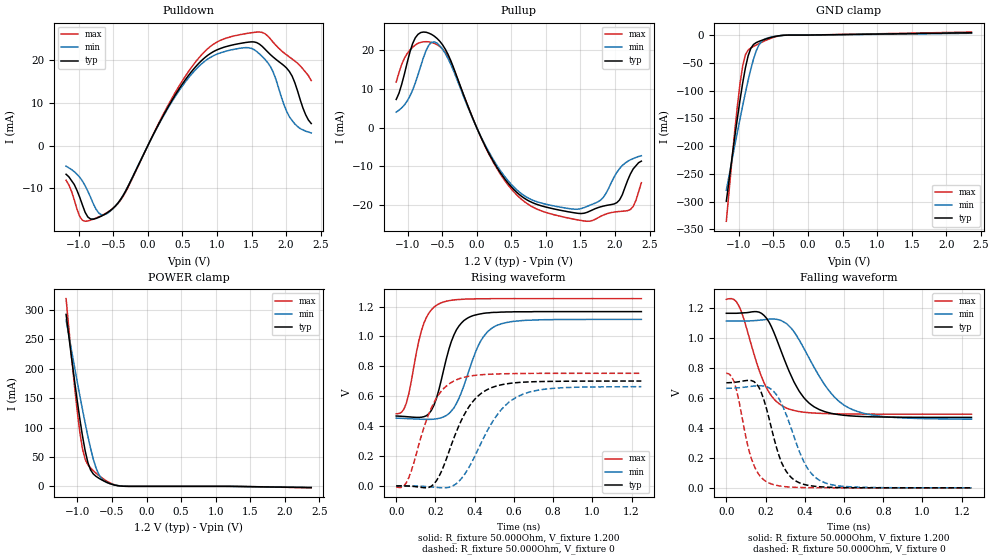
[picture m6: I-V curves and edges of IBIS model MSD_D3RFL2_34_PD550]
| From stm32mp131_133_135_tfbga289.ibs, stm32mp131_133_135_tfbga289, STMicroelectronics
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[Model] MSD_D3RFL2_34_PD550
Model_type   I/O
C_comp 2.431pF   2.345pF   2.556pF
Vinh = 820.000mV
Vinl = 380.000mV
Vmeas = 600.000mV
Vref = 600.000mV
[Model Spec]
Vinh   820.000mV   790.000mV   870.000mV
Vinl   380.000mV   350.000mV   430.000mV
Vmeas   600.000mV   570.000mV   650.000mV
Vref   600.000mV   570.000mV   650.000mV
[Receiver Thresholds]
Vth   =  0.600V
Vth_min  =  0.5880V
Vth_max  =  0.6120V
Vinh_ac  =  0.220V
Vinh_dc  =  0.130V
Vinl_ac  = -0.220V
Vinl_dc  = -0.130V
Tslew_ac =  5.000ns |Not specified, so set to high value
[Temperature Range]   25.000   125.000   -40.000
[Voltage Range]   1.200V   1.140V   1.300V
[GND Clamp Reference]   0.00V   0.00V   0.00V
[Pulldown Reference]   0.00V   0.00V   0.00V
[POWER Clamp Reference]   1.200V   1.140V   1.300V
[Pullup Reference]   1.200V   1.140V   1.300V
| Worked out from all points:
|   slope of the pulldown table from 0 to 0.18 V, typ, clamps not added: 31.3 ohm
|   slope of the pullup table from 0 to 0.18 V, typ, clamps not added: 26.5 ohm
|   GND clamp passes 1 mA (typ) near -0.40 V on its own axis
|   POWER clamp passes 1 mA (typ) near -0.41 V on its own axis
|   rising waveform, R_fixture 50.000Ohm, V_fixture 1.200: 20-80 % time 90.7ps typ, 117ps min, 77.4ps max; typ from 0.468 V to 1.17 V
|   rising waveform, R_fixture 50.000Ohm, V_fixture 0: 20-80 % time 145ps typ, 176ps min, 124ps max; typ from 0.001 V to 0.702 V
|   falling waveform, R_fixture 50.000Ohm, V_fixture 1.200: 20-80 % time 145ps typ, 191ps min, 120ps max; typ from 1.17 V to 0.47 V
|   falling waveform, R_fixture 50.000Ohm, V_fixture 0: 20-80 % time 94.7ps typ, 121ps min, 80.9ps max; typ from 0.701 V to 0 V
[GND Clamp]
-1.182V   -299.4mA   -279.4mA   -335.5mA
-1.064V   -187.2mA   -201.7mA   -177.2mA
-984.9mV  -117.7mA   -151.5mA   -88.38mA
-945.5mV  -86.38mA   -127.3mA   -55.57mA
-906.1mV  -58.98mA   -103.8mA   -35.45mA
-866.7mV  -37.48mA   -81.61mA   -27.05mA
-787.9mV  -16.83mA   -42.88mA   -20.43mA
-709.1mV  -11.34mA   -17.45mA   -15.32mA
-630.3mV  -7.809mA   -7.49mA    -10.62mA
-512.1mV  -3.532mA   -3.013mA   -4.68mA
-315.1mV  -161.1uA   -227.4uA   -151.1uA
2.364V    4.162mA    3.192mA    5.446mA
[Power Clamp]
-1.164V   292.2mA    282.4mA    319.1mA
-1.085V   218.5mA    230.7mA    219.9mA
-1.006V   148.3mA    179.9mA    131mA
-966.7mV  115.8mA    155mA      93.19mA
-927.3mV  85.99mA    130.7mA    63.83mA
-887.9mV  60.26mA    107.3mA    45.72mA
-809.1mV  27.71mA    64.21mA    31.02mA
-730.3mV  16.94mA    31.06mA    22.31mA
-690.9mV  13.86mA    20.24mA    18.46mA
-572.7mV  6.594mA    6.506mA    8.718mA
-336.4mV  182.6uA    351.4uA    213.2uA
2.382V    -2.141mA   -1.766mA   -2.539mA
[Pulldown]
-1.182V   -6.7mA     -4.8mA     -8.1mA
-945.5mV  -13.91mA   -8.3mA     -17.51mA
-827.3mV  -17.2mA    -12.13mA   -17.46mA
-709.1mV  -16.81mA   -15.79mA   -16.7mA
-590.9mV  -15.77mA   -15.93mA   -15.7mA
-354.6mV  -11.63mA   -11.57mA   -11.83mA
590.9mV   16.52mA    15.97mA    17.46mA
906.1mV   21.65mA    20.73mA    23.3mA
1.261V    23.76mA    22.65mA    25.8mA
1.733V    22.01mA    19.52mA    25.76mA
2.009V    18.19mA    8.04mA     21.29mA
2.364V    5.2mA      3mA        15.3mA
[Pullup]
-1.164V   7.3mA      4.009mA    11.8mA
-887.9mV  23.28mA    11.57mA    21.42mA
-730.3mV  24.71mA    20.07mA    22.27mA
-612.1mV  23.69mA    22.22mA    21.84mA
-375.8mV  17.4mA     16.45mA    16.97mA
215.2mV   -7.946mA   -7.529mA   -8.168mA
727.3mV   -18.74mA   -18.09mA   -19.68mA
1.515V    -22.28mA   -20.97mA   -24.1mA
1.791V    -20.54mA   -18.82mA   -23.03mA
1.988V    -19.79mA   -12.79mA   -21.91mA
2.224V    -12mA      -8.343mA   -21.22mA
2.382V    -8.7mA     -7.295mA   -14.29mA
[Ramp]
R_load=50.000Ohm
dV/dt_r   419.370mV/118.000ps  396.479mV/147.000ps  454.470mV/101.000ps
dV/dt_f   419.370mV/121.000ps  396.449mV/157.000ps  454.470mV/100.500ps
[Rising waveform]
R_fixture=50.000Ohm
V_fixture=1.200
V_fixture_min=1.140
V_fixture_max=1.300
0s        468.1mV    453.9mV    482.9mV
52ps      463.9mV    451.1mV    555.1mV
141ps     463.3mV    446mV      1.088V
179ps     505.2mV    446.1mV    1.178V
218ps     645.6mV    452.7mV    1.218V
269ps     916.2mV    484.1mV    1.239V
320ps     1.07V      586.7mV    1.247V
422ps     1.149V     948.3mV    1.252V
511ps     1.161V     1.073V     1.253V
1.25ns    1.166V     1.114V     1.253V
[Rising waveform]
R_fixture=50.000Ohm
V_fixture=0
0s        902.8uV    884.2uV    -6.476mV
64ps      -166.2uV   774uV      55.98mV
179ps     -1.324mV   -6.145mV   522.1mV
230ps     96.19mV    -11.52mV   634.6mV
294ps     320.6mV    4.828mV    702.6mV
409ps     592.2mV    222mV      741mV
524ps     673.2mV    492.4mV    749.7mV
613ps     691mV      594.3mV    752mV
792ps     699.7mV    652.2mV    753.4mV
1.25ns    701.9mV    664.2mV    753.6mV
[Falling waveform]
R_fixture=50.000Ohm
V_fixture=1.200
V_fixture_min=1.140
V_fixture_max=1.300
0s        1.165V     1.113V     1.258V
64ps      1.166V     1.113V     1.215V
192ps     1.151V     1.122V     701.8mV
243ps     1.036V     1.127V     592.6mV
307ps     819.6mV    1.096V     532.3mV
422ps     565.5mV    865.9mV    501.4mV
524ps     500.7mV    647.6mV    495.1mV
626ps     480.9mV    532.6mV    492.7mV
830ps     472.1mV    472.4mV    491.7mV
1.25ns    470mV      458.2mV    491.6mV
[Falling waveform]
R_fixture=50.000Ohm
V_fixture=0
0s        701.3mV    664.1mV    764.5mV
39ps      704mV      665.9mV    709.5mV
141ps     709.1mV    679.3mV    149mV
179ps     633.5mV    681.2mV    67.44mV
218ps     462.5mV    667.3mV    31.96mV
269ps     213.1mV    593.9mV    13.09mV
320ps     84.51mV    437.1mV    5.624mV
409ps     18.81mV    140.9mV    1.3mV
486ps     6.418mV    42.86mV    365.1uV
1.25ns    2.255uV    24.79uV    691.5nV
